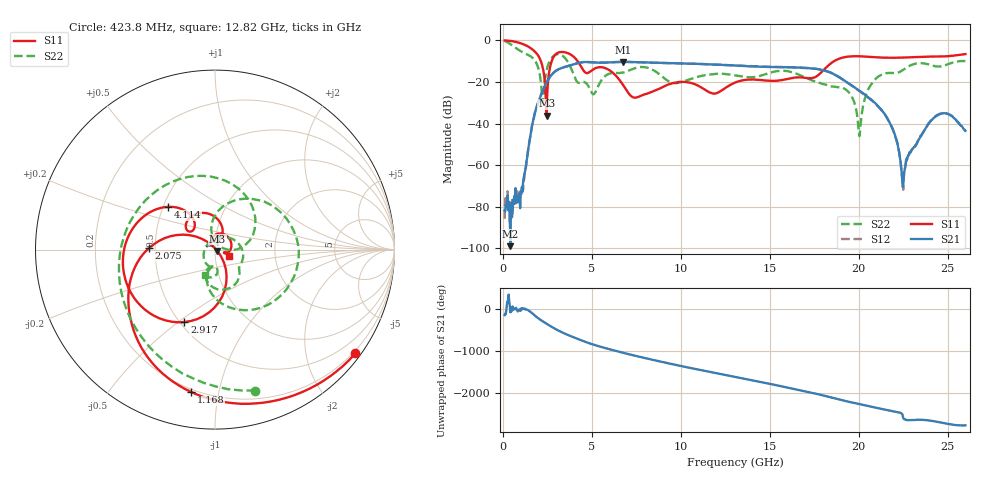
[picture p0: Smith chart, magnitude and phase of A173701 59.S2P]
!  2-Port S-parameters saved by WinCal
! VAR MeasName=S-Parameters (CALIBRATED_DATA) read from VNA (N5245A)
! VAR MeasDate=2017-6-7 10:32:20
! VAR NAME=A173701 59
! VAR FILENAME=A173701 59.S2P
! VAR DATE=2017-6-7 10:32:20
! VAR PHYS_PORTS=1,2
# Hz S DB R 50
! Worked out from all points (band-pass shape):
!   801 points, 100 MHz to 26 GHz, reference 50 ohm
!   highest |S21| = -10.32 dB at 6.769 GHz (marker M1); lowest = -99.1 dB at 423.8 MHz (marker M2)
!   |S21| within 3 dB of the highest: 3.288 GHz to 17.15 GHz (13.86 GHz wide, 136 % of centre)
!   lowest |S11| = -36.3 dB at 2.463 GHz (marker M3), VSWR 1.03, Z = 51.3 - j0.776 ohm
!   |S11| at or under -10 dB: 2.139 GHz to 2.746 GHz (606.6 MHz wide, 24.8 % of centre); 4.206 GHz to 18.61 GHz (14.41 GHz wide, 126 % of centre)
!   |S22| runs from -46.1 to -0.2 dB; largest |S21 - S12| = 0.0036
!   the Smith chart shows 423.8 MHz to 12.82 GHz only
!   S11 on the Smith chart (normalised r, x): 423.8 MHz: 0.14, -3.03; 1.168 GHz: 0.18, -0.83; 2.075 GHz: 0.46, +0.01; 2.917 GHz: 0.53, -0.53; 4.114 GHz: 0.53, +0.29; 12.82 GHz: 1.17, -0.08
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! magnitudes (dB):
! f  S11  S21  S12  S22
! 100 MHz  0.0  -81.9  -85.8  -0.2
! 423.8 MHz  -0.2  -99.1  -84.9  -1.8
! 1.168 GHz  -1.9  -66.2  -67.2  -5.9
! 2.075 GHz  -8.7  -27.9  -27.9  -16.3
! 2.269 GHz  -14.1  -23.7  -23.7  -28.2
! 2.463 GHz  -36.3  -20.2  -20.2  -14.2
! 2.917 GHz  -7.2  -15.1  -15.0  -7.1
! 4.114 GHz  -9.0  -11.2  -11.2  -19.1
! 4.438 GHz  -13.2  -10.5  -10.5  -20.0
! 5.118 GHz  -13.7  -10.6  -10.6  -25.9
! 6.769 GHz  -21.6  -10.3  -10.4  -15.5
! 8.744 GHz  -23.5  -10.8  -10.8  -15.9
! 12.82 GHz  -21.3  -11.9  -12.0  -16.5
! 13.05 GHz  -20.3  -12.1  -12.1  -16.8
! 17.39 GHz  -18.1  -13.5  -13.4  -19.3
! 19.36 GHz  -7.8  -20.3  -20.3  -24.3
! 20.04 GHz  -7.6  -24.3  -24.4  -46.1
! 20.63 GHz  -7.9  -27.9  -28.1  -22.2
! 21.69 GHz  -8.3  -38.8  -38.8  -15.7
! 22.5 GHz  -8.2  -70.5  -71.9  -14.2
! 24.32 GHz  -7.8  -36.6  -36.5  -12.5
! 26 GHz  -6.6  -43.5  -43.6  -10.0
